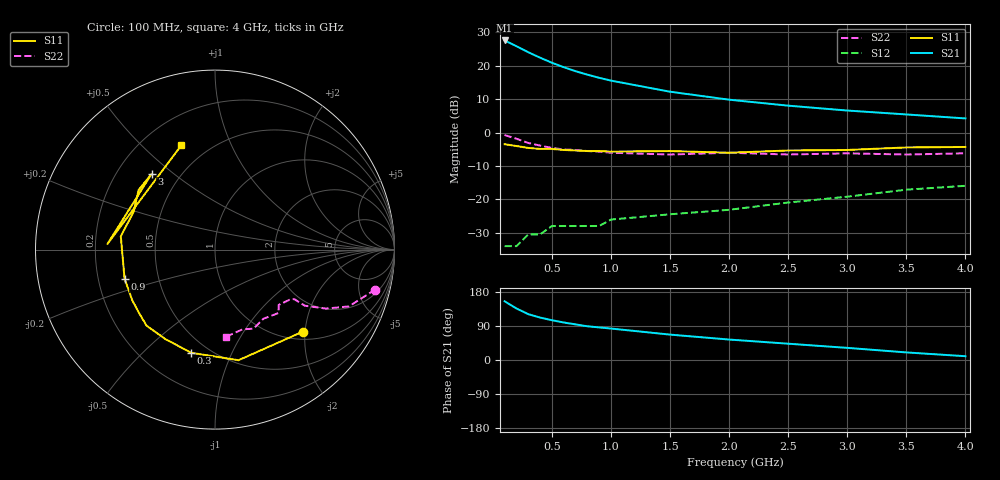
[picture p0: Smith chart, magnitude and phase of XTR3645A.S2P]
! HXTR-3645 Common Emitter
! Vce=10V  Ic=10mA
# ghz s ma r 50
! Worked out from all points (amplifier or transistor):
!   16 points, 100 MHz to 4 GHz, reference 50 ohm
!   highest |S21| = 27.6 dB at 100 MHz (marker M1)
!   |S21| within 3 dB of that: start of sweep to 270.9 MHz
!   unconditionally stable (mu >= 1): 1.456 GHz to 2.984 GHz
!   at 300 MHz: K = 0.35, MSG = 27.3 dB, |S12| = -30.5 dB
!   at 900 MHz: K = 0.88, MSG = 22.2 dB, |S12| = -28.0 dB
!   at 4 GHz: K = 0.81, MSG = 10.1 dB, |S12| = -15.9 dB
!   lowest NFmin = 1.20 dB at 1 GHz
!   S11 on the Smith chart (normalised r, x): 100 MHz: 1.18, -1.95; 300 MHz: 0.40, -0.71; 900 MHz: 0.31, -0.14; 3 GHz: 0.35, +0.42; 4 GHz: 0.36, +0.66
0.1  0.67 -43.0  23.92 155.0  0.02 66.0  0.92 -14.0
0.2  0.63 -78.0  19.63 136.0  0.02 70.0  0.81 -23.0
0.3  0.59 -103.0  15.94 121.0  0.03 53.0  0.7 -28.0
0.4  0.57 -119.0  13.22 112.0  0.03 52.0  0.64 -30.0
0.5  0.57 -132.0  11.11 105.0  0.04 46.0  0.59 -32.0
0.6  0.55 -141.0  9.52 99.0  0.04 49.0  0.56 -32.0
0.7  0.54 -149.0  8.3 94.0  0.04 50.0  0.55 -32.0
0.8  0.53 -156.0  7.37 89.0  0.04 49.0  0.53 -32.0
0.9  0.53 -162.0  6.61 86.0  0.04 51.0  0.52 -32.0
1  0.52 -168.0  6 83.0  0.05 50.0  0.5 -34.0
1.5  0.53 172.0  4.09 67.0  0.06 55.0  0.47 -41.0
2  0.5 155.0  3.11 54.0  0.07 58.0  0.5 -45.0
2.5  0.54 142.0  2.53 43.0  0.09 59.0  0.47 -55.0
3  0.55 130.0  2.14 32.0  0.11 58.0  0.49 -64.0
3.5  0.6 177.0  1.87 20.0  0.14 56.0  0.47 -71.0
4  0.61 108.0  1.63 10.0  0.16 52.0  0.49 -83.0
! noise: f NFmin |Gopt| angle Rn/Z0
1  1.2  0.2  135  0.146
2  1.9  0.39  -177  0.044
